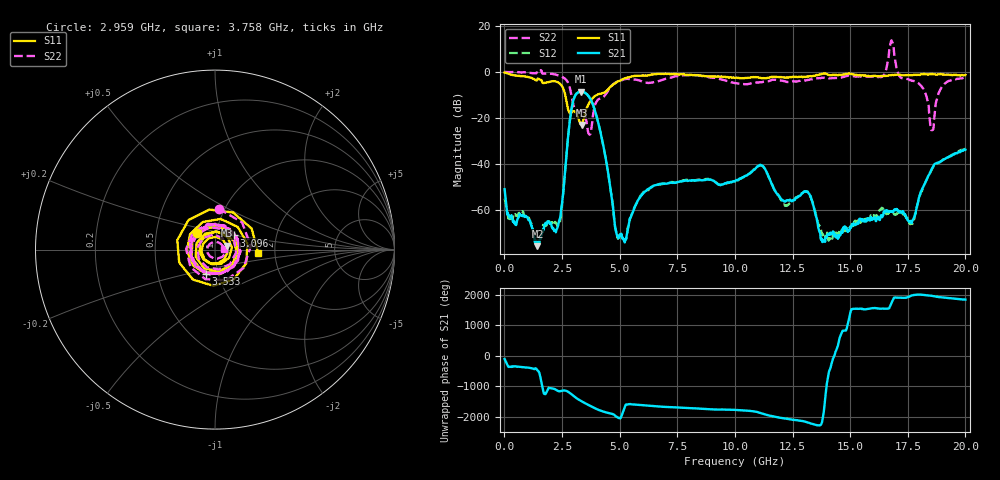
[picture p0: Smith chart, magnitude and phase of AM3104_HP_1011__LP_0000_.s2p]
!Created with skrf (http://scikit-rf.org).
# Hz S RI R 50.0
!freq ReS11 ImS11 ReS21 ImS21 ReS12 ImS12 ReS22 ImS22
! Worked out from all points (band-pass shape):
!   1601 points, 10 MHz to 20 GHz, reference 50 ohm
!   highest |S21| = -8.59 dB at 3.321 GHz (marker M1); lowest = -75.9 dB at 1.434 GHz (marker M2)
!   |S21| within 3 dB of the highest: 3.019 GHz to 3.723 GHz (704.7 MHz wide, 20.9 % of centre)
!   lowest |S11| = -23.1 dB at 3.346 GHz (marker M3), VSWR 1.15, Z = 57.1 + j2.46 ohm
!   |S11| at or under -10 dB: 2.64 GHz to 4.027 GHz (1.388 GHz wide, 41.6 % of centre)
!   |S22| runs from -27.3 to 13.7 dB; largest |S21 - S12| = 0.015
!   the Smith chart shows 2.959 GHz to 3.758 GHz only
!   S11 on the Smith chart (normalised r, x): 2.959 GHz: 0.80, +0.15; 3.096 GHz: 1.22, +0.19; 3.533 GHz: 0.87, -0.24; 3.758 GHz: 1.63, -0.06
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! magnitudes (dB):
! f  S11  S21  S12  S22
! 10 MHz  -0.2  -51.1  -55.2  0.0
! 1.434 GHz  -3.2  -75.9  -74.8  0.7
! 2.396 GHz  -5.0  -64.3  -65.8  -1.7
! 2.959 GHz  -17.2  -13.7  -13.7  -12.8
! 3.096 GHz  -17.7  -9.9  -9.9  -16.9
! 3.321 GHz  -22.9  -8.6  -8.7  -16.9
! 3.346 GHz  -23.1  -8.6  -8.7  -17.0
! 3.533 GHz  -16.8  -9.4  -9.4  -20.2
! 3.758 GHz  -12.4  -12.3  -12.3  -25.8
! 4.933 GHz  -4.1  -72.0  -72.7  -4.2
! 6.682 GHz  -0.9  -49.1  -49.0  -4.1
! 10.01 GHz  -2.6  -47.6  -47.7  -4.9
! 11.14 GHz  -2.7  -40.7  -40.8  -4.5
! 12.17 GHz  -2.5  -56.5  -58.2  -4.1
! 13.34 GHz  -1.9  -55.9  -56.0  -3.2
! 13.82 GHz  -0.8  -73.5  -70.7  -2.6
! 16.35 GHz  -1.8  -62.7  -59.8  -2.3
! 16.68 GHz  -1.5  -61.0  -61.4  7.2
! 17.69 GHz  -1.5  -64.9  -66.2  -3.9
! 18.55 GHz  -0.9  -42.1  -42.3  -25.4
! 18.99 GHz  -1.1  -38.7  -38.5  -6.5
! 20 GHz  -1.4  -33.9  -33.5  -2.5
